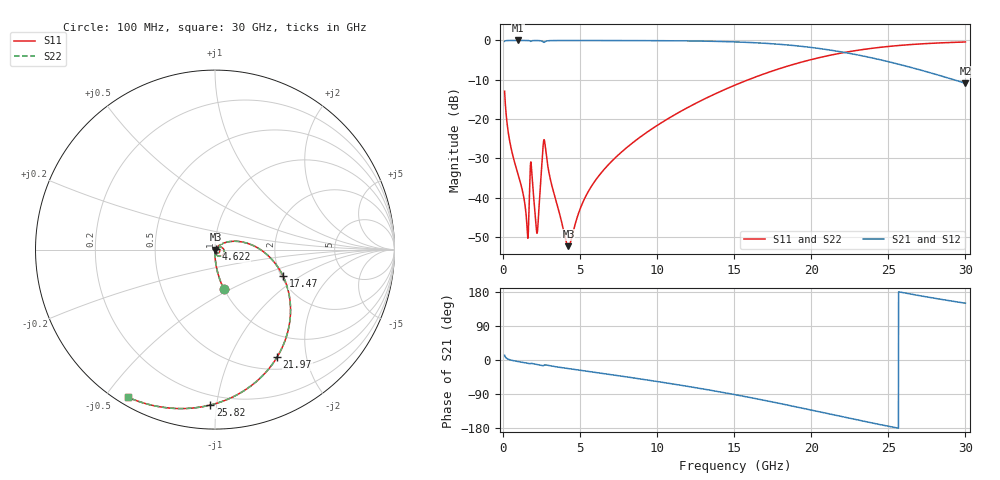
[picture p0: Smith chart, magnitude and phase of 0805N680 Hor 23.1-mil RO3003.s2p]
# GHz S MA R 50
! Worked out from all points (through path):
!   3201 points, 100 MHz to 30 GHz, reference 50 ohm
!   highest |S21| = -0.01 dB at 978.3 MHz (marker M1); lowest = -10.9 dB at 30 GHz (marker M2)
!   group delay of S21, straight-line fit = 20.3 ps
!   lowest |S11| = -52.4 dB at 4.239 GHz (marker M3), VSWR 1.00, Z = 50.2 - j0.086 ohm
!   |S11| at or under -10 dB: start of sweep to 15.92 GHz
!   |S22| runs from -52.4 to -0.4 dB; largest |S21 - S12| = 0
!   S11 on the Smith chart (normalised r, x): 100 MHz: 1.00, -0.46; 4.622 GHz: 1.01, +0.00; 17.47 GHz: 2.05, -0.73; 21.97 GHz: 0.66, -1.52; 25.82 GHz: 0.14, -0.96; 30 GHz: 0.03, -0.57
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0.1  0.2255 -77.4  0.9739 12.5  0.9739 12.5  0.2255 -77.4
0.4457187  0.05033 -88.9  0.9982 0.5  0.9982 0.5  0.05033 -88.9
0.9783125  0.01958 -91.8  0.999 -4.1  0.999 -4.1  0.01958 -91.8
1.538938  0.004694 -74.9  0.9981 -8.0  0.9981 -8.0  0.004694 -74.9
1.865969  0.02013 -64.4  0.9883 -9.1  0.9883 -9.1  0.02013 -64.4
2.202344  0.003506 -20.7  0.9965 -11.8  0.9965 -11.8  0.003506 -20.7
2.314469  0.006515 30.7  0.9952 -12.7  0.9952 -12.7  0.006515 30.7
2.56675  0.03754 20.1  0.969 -15.0  0.969 -15.0  0.03754 20.1
2.706906  0.05015 -45.1  0.9571 -13.0  0.9571 -13.0  0.05015 -45.1
3.155406  0.01448 -87.5  0.9952 -16.1  0.9952 -16.1  0.01448 -87.5
4.239281  0.002408 -20.8  0.9974 -22.6  0.9974 -22.6  0.002408 -20.8
4.622375  0.004173 31.0  0.9975 -24.8  0.9975 -24.8  0.004173 31.0
5.089563  0.007943 45.4  0.9974 -27.5  0.9974 -27.5  0.007943 45.4
6.864875  0.02659 46.7  0.9969 -37.8  0.9969 -37.8  0.02659 46.7
10.06978  0.08452 30.6  0.9928 -57.2  0.9928 -57.2  0.08452 30.6
15.05  0.27 -2.5  0.9575 -91.4  0.9575 -91.4  0.27 -2.5
17.47003  0.408 -21.4  0.9067 -110.6  0.9067 -110.6  0.408 -21.4
20.03956  0.5733 -43.2  0.8119 -132.6  0.8119 -132.6  0.5733 -43.2
21.97372  0.6924 -60.1  0.7133 -149.5  0.7133 -149.5  0.6924 -60.1
25.01978  0.8386 -85.5  0.5355 -175.0  0.5355 -175.0  0.8386 -85.5
25.82334  0.8667 -91.8  0.4892 178.8  0.4892 178.8  0.8667 -91.8
30  0.9551 -120.6  0.2847 149.9  0.2847 149.9  0.9551 -120.6
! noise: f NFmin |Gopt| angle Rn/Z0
0.1  0.0004265  0.859  0.6918  0.0006476
3.417  0.007977  0.7581  18.31  0.006508
6.743  0.009915  0.6467  35.51  0.004848
10.06  0.01359  0.6289  51.74  0.005629
13.39  0.0178  0.6328  66.93  0.006483
16.7  0.02289  0.6505  81.06  0.007425
20.03  0.02945  0.6793  94.41  0.008543
23.35  0.03836  0.7178  107.2  0.009936
26.67  0.05133  0.7645  119.8  0.01171
30  0.0715  0.8164  132.6  0.01386
